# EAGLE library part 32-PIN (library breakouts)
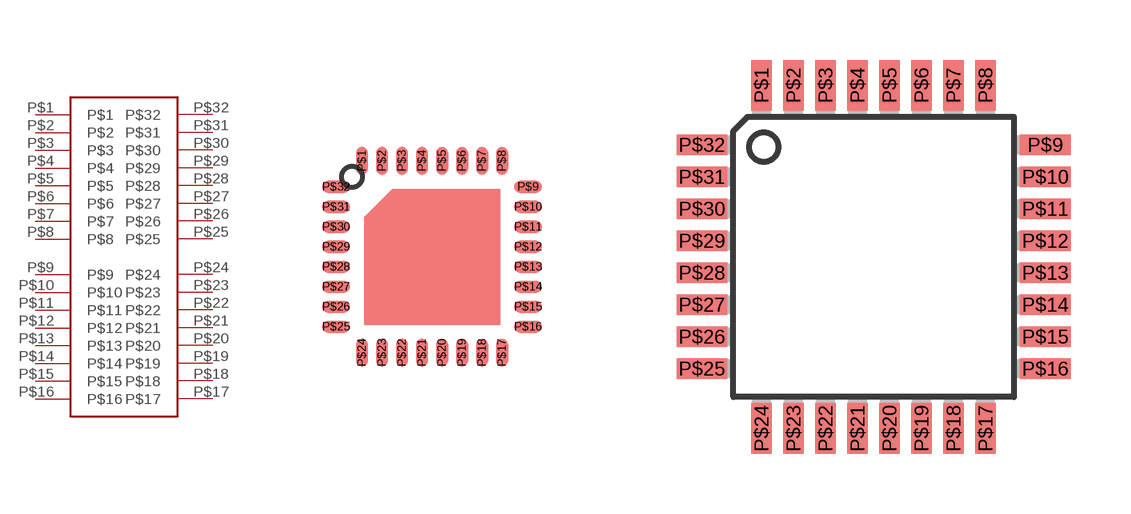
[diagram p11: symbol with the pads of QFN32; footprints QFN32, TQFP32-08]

Designator prefix -

## 32-PINQFN  [QFN32]
P$1  P$1
P$2  P$2
P$3  P$3
P$4  P$4
P$5  P$5
P$6  P$6
P$7  P$7
P$8  P$8
P$9  P$9
P$10  P$10
P$11  P$11
P$12  P$12
P$13  P$13
P$14  P$14
P$15  P$15
P$16  P$16
P$17  P$17
P$18  P$18
P$19  P$19
P$20  P$20
P$21  P$21
P$22  P$22
P$23  P$23
P$24  P$24
P$25  P$25
P$26  P$26
P$27  P$27
P$28  P$28
P$29  P$29
P$30  P$30
P$31  P$31
P$32  P$32

## 32-PINTQFP  [TQFP32-08]
Pads as for QFN32

## Footprint QFN32 (pad centres in mm)
smd 0.3 x 0.7: P$1 -1.75,2.4; P$2 -1.25,2.4; P$3 -0.75,2.4; P$4 -0.25,2.4; P$5 0.25,2.4; P$6 0.75,2.4; P$7 1.25,2.4; P$8 1.75,2.4; P$17 1.75,-2.4; P$18 1.25,-2.4; P$19 0.75,-2.4; P$20 0.25,-2.4; P$21 -0.25,-2.4; P$22 -0.75,-2.4; P$23 -1.25,-2.4; P$24 -1.75,-2.4
smd 0.7 x 0.3: P$9 2.4,1.75; P$10 2.4,1.25; P$11 2.4,0.75; P$12 2.4,0.25; P$13 2.4,-0.25; P$14 2.4,-0.75; P$15 2.4,-1.25; P$16 2.4,-1.75; P$25 -2.4,-1.75; P$26 -2.4,-1.25; P$27 -2.4,-0.75; P$28 -2.4,-0.25; P$29 -2.4,0.25; P$30 -2.4,0.75; P$31 -2.4,1.25; P$32 -2.4,1.75

## Footprint TQFP32-08 (pad centres in mm)
Thin Plasic Quad Flat Package Grid 0.8 mm
smd 0.508 x 1.27: P$1 -2.8,4.293; P$2 -2,4.293; P$3 -1.2,4.293; P$4 -0.4,4.293; P$5 0.4,4.293; P$6 1.2,4.293; P$7 2,4.293; P$8 2.8,4.293; P$17 2.8,-4.293; P$18 2,-4.293; P$19 1.2,-4.293; P$20 0.4,-4.293; P$21 -0.4,-4.293; P$22 -1.2,-4.293; P$23 -2,-4.293; P$24 -2.8,-4.293
smd 1.27 x 0.508: P$9 4.293,2.8; P$10 4.293,2; P$11 4.293,1.2; P$12 4.293,0.4; P$13 4.293,-0.4; P$14 4.293,-1.2; P$15 4.293,-2; P$16 4.293,-2.8; P$25 -4.293,-2.8; P$26 -4.293,-2; P$27 -4.293,-1.2; P$28 -4.293,-0.4; P$29 -4.293,0.4; P$30 -4.293,1.2; P$31 -4.293,2; P$32 -4.293,2.8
